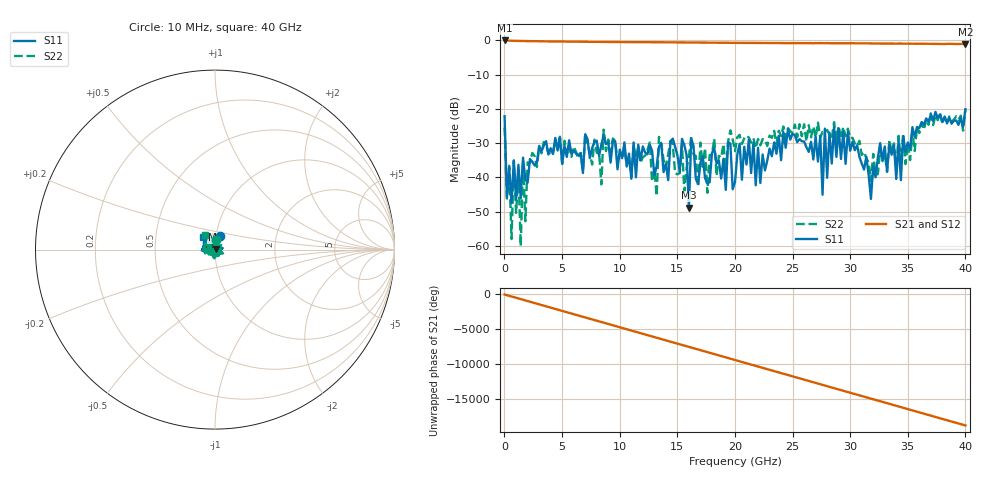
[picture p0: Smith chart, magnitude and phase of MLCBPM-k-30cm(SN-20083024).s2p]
!Keysight Technologies,N5225A,MY51451228,A.10.40.14
!Date: Friday, November 20, 2020 11:37:39
!Correction: S11(Full 2 Port(1,2))
!S21(Full 2 Port(1,2))
!S12(Full 2 Port(1,2))
!S22(Full 2 Port(1,2))
!S2P File: Measurements: S11, S21, S12, S22:
# Hz S  dB  R 50
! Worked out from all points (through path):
!   201 points, 10 MHz to 40 GHz, reference 50 ohm
!   highest |S21| = -0.02 dB at 10 MHz (marker M1); lowest = -1.1 dB at 40 GHz (marker M2)
!   lowest |S11| = -48.9 dB at 16.01 GHz (marker M3), VSWR 1.01, Z = 50.3 + j0.122 ohm
!   |S11| at or under -10 dB: start of sweep to end of sweep
!   |S22| runs from -60.1 to -20.1 dB; largest |S21 - S12| = 0.012
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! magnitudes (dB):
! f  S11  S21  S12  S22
! 10 MHz  -22.1  0.0  -0.1  -25.4
! 209.9 MHz  -45.8  0.0  0.0  -46.2
! 409.9 MHz  -37.1  -0.1  -0.1  -36.6
! 609.9 MHz  -47.5  -0.1  -0.1  -58.0
! 809.8 MHz  -35.1  -0.1  -0.1  -35.1
! 1.21 GHz  -36.3  -0.2  -0.1  -38.2
! 1.41 GHz  -46.1  -0.2  -0.2  -60.1
! 1.61 GHz  -34.2  -0.2  -0.2  -35.2
! 1.81 GHz  -40.6  -0.2  -0.2  -52.8
! 3.409 GHz  -30.7  -0.3  -0.3  -29.7
! 6.808 GHz  -38.7  -0.4  -0.4  -38.2
! 12.61 GHz  -30.5  -0.5  -0.5  -29.8
! 13.21 GHz  -36.7  -0.5  -0.5  -45.5
! 13.41 GHz  -31.1  -0.5  -0.6  -28.2
! 15.41 GHz  -28.8  -0.6  -0.6  -30.6
! 16.01 GHz  -48.9  -0.6  -0.6  -34.0
! 16.21 GHz  -28.6  -0.6  -0.6  -28.1
! 17.61 GHz  -41.7  -0.6  -0.6  -44.5
! 20 GHz  -41.4  -0.7  -0.7  -32.3
! 26.8 GHz  -34.8  -0.8  -0.8  -25.1
! 33.4 GHz  -30.5  -0.9  -0.9  -29.0
! 40 GHz  -20.1  -1.1  -1.1  -20.1
